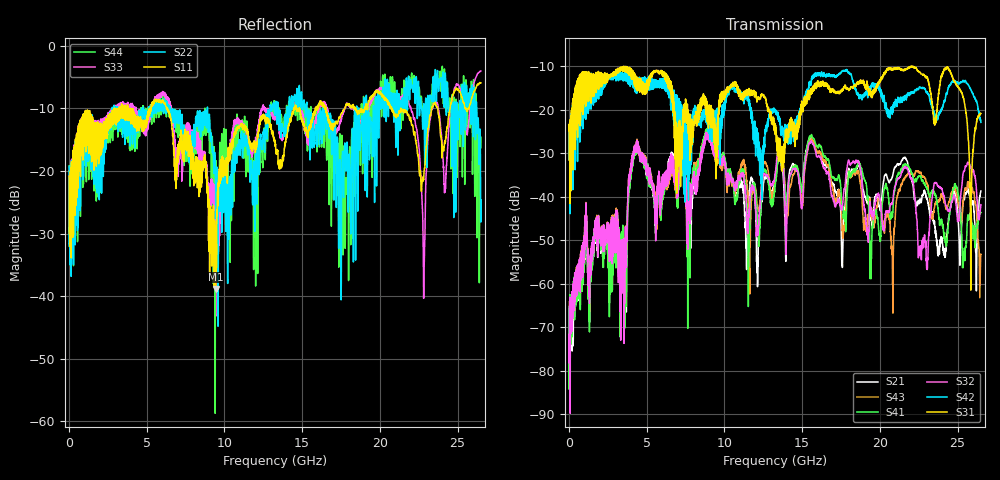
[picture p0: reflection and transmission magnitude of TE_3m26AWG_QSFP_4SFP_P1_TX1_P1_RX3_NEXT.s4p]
!Agilent Technologies,N5222A,MY51421691,A.10.00.00
!Agilent N5222A: A.10.00.00
!Date: Friday, January 30, 2015 12:34:27
!Correction: S11(Full 4 Port(1,2,3,4))
!S12(Full 4 Port(1,2,3,4))
!S13(Full 4 Port(1,2,3,4))
!S14(Full 4 Port(1,2,3,4))
!S21(Full 4 Port(1,2,3,4))
!S22(Full 4 Port(1,2,3,4))
!S23(Full 4 Port(1,2,3,4))
!S24(Full 4 Port(1,2,3,4))
!S31(Full 4 Port(1,2,3,4))
!S32(Full 4 Port(1,2,3,4))
!S33(Full 4 Port(1,2,3,4))
!S34(Full 4 Port(1,2,3,4))
!S41(Full 4 Port(1,2,3,4))
!S42(Full 4 Port(1,2,3,4))
!S43(Full 4 Port(1,2,3,4))
!S44(Full 4 Port(1,2,3,4))
!S4P File: Measurements: <S11,S12,S13,S14>,
!<S21,S22,S23,S24>,
!<S31,S32,S33,S34>,
!<S41,S42,S43,S44>:
# Hz S  dB  R 50.0
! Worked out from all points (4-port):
!   2650 points, 10 MHz to 26.5 GHz, reference 50 ohm
!   strongest paths, dB at 10 MHz, 6.63 GHz, 13.26 GHz, 19.88 GHz, 26.5 GHz:
!     S31: -24.8, -18.2, -24.4, -13.7, -20.8
!     S42: -24.9, -15.7, -19.9, -14.1, -22.9
!     S32: -71.7, -30.4, -34.9, -39.3, -41.8
!     S41: -65.3, -30.6, -37.2, -45.4, -43.6
!     S43: -73.6, -31.1, -36.2, -40.6, -53.2
!     S21: -66.1, -29.8, -36.4, -40.6, -38.7
!   lowest |S11| = -38.9 dB at 9.43 GHz (marker M1), VSWR 1.02, Z = 50.5 + j1.03 ohm
!   |S11| at or under -10 dB: start of sweep to 2.939 GHz; 6.342 GHz to 14.46 GHz (8.115 GHz wide, 78 % of centre); 21.35 GHz to 23.34 GHz (1.989 GHz wide, 8.9 % of centre)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
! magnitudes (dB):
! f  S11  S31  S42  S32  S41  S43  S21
! 10 MHz  -20.8  -24.8  -24.9  -71.7  -65.3  -73.6  -66.1
! 3.61 GHz  -10.4  -10.7  -12.0  -57.1  -70.2  -58.0  -69.6
! 4.3 GHz  -11.2  -12.9  -13.8  -28.4  -29.0  -28.4  -29.0
! 9.43 GHz  -38.9  -27.5  -20.1  -30.2  -28.0  -30.2  -28.0
! 12.16 GHz  -13.8  -17.2  -30.8  -48.4  -46.8  -42.8  -56.0
! 22.81 GHz  -21.4  -11.8  -15.1  -50.2  -37.0  -35.5  -39.4
! 26.5 GHz  -5.9  -20.8  -22.9  -41.8  -43.6  -53.2  -38.7
